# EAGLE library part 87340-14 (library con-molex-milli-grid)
RECEPTACAL
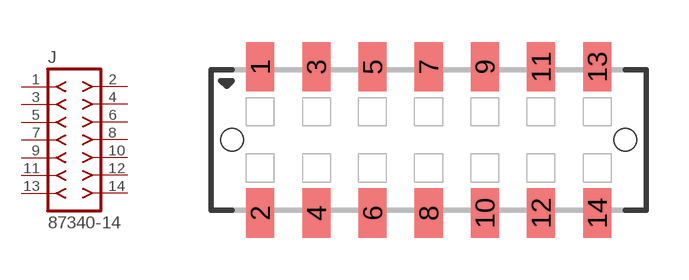
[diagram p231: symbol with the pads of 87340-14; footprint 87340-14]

Designator prefix J

## 87340-14  [87340-14]
1  1  pas
2  2  pas
3  3  pas
4  4  pas
5  5  pas
6  6  pas
7  7  pas
8  8  pas
9  9  pas
10  10  pas
11  11  pas
12  12  pas
13  13  pas
14  14  pas

## Footprint 87340-14 (pad centres in mm)
RECEPTACAL SMD Dual Row, Vertical, Low Profile
smd 1 x 1.75: 1 -6,2.6; 2 -6,-2.6; 3 -4,2.6; 4 -4,-2.6; 5 -2,2.6; 6 -2,-2.6; 7 0,2.6; 8 0,-2.6; 9 2,2.6; 10 2,-2.6; 11 4,2.6; 12 4,-2.6; 13 6,2.6; 14 6,-2.6
hole 0.8 at -7,0
hole 0.8 at 7,0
